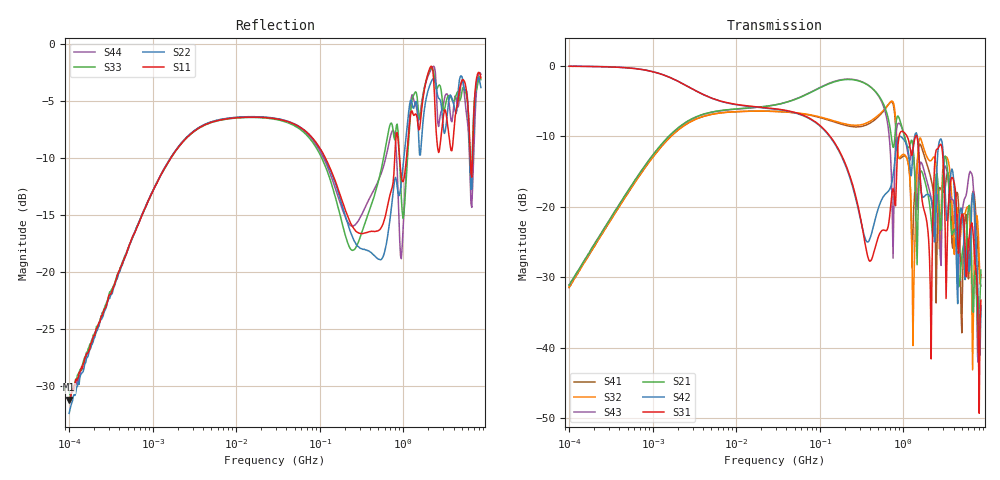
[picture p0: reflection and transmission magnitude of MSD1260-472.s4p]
# MHz S MA R 50
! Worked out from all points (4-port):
!   498 points, 100 kHz to 8.5 GHz, reference 50 ohm
!   strongest paths, dB at 100 kHz, 1.698 MHz, 29.49 MHz, 500.7 MHz, 8.5 GHz:
!     S31: -0.1, -1.8, -6.1, -24.3, -33.3
!     S42: -0.1, -1.8, -6.2, -20.3, -34.4
!     S21: -31.1, -9.6, -5.5, -4.1, -29.0
!     S43: -31.1, -9.6, -5.5, -4.2, -34.0
!     S32: -31.4, -9.9, -6.5, -7.0, -29.6
!     S41: -31.5, -9.9, -6.5, -7.3, -31.2
!   lowest |S11| = -31.2 dB at 100 kHz (marker M1), VSWR 1.06, Z = 50 + j2.77 ohm
!   |S11| at or under -10 dB: 117.4 MHz to 790.6 MHz (673.2 MHz wide, 148 % of centre); 903.2 MHz to 1.092 GHz (188.6 MHz wide, 18.9 % of centre); 6.36 GHz to 6.737 GHz (377 MHz wide, 5.76 % of centre)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
0.1  0.02766 88.8  0.02777 85.4  0.9921 -1.6  0.02665 -95.1
     0.02777 85.4  0.02411 88.8  0.02698 -95.0  0.9938 -1.6
     0.9921 -1.6  0.02698 -95.0  0.03029 90.1  0.02801 84.4
     0.02665 -95.1  0.9938 -1.6  0.02801 84.4  0.02776 92.2
3.607286  0.4304 26.0  0.4429 28.3  0.6464 -20.5  0.4275 -155.2
          0.4429 28.3  0.4324 26.1  0.4275 -155.4  0.6456 -20.8
          0.6464 -20.5  0.4275 -155.4  0.4297 26.0  0.4421 28.4
          0.4275 -155.2  0.6456 -20.8  0.4421 28.4  0.4324 26.2
241.0775  0.1616 -48.8  0.7984 -37.0  0.1513 -131.4  0.3705 49.2
          0.7984 -37.0  0.1462 -55.2  0.38 45.5  0.1463 -133.8
          0.1513 -131.4  0.38 45.5  0.1253 -31.4  0.8027 -39.9
          0.3705 49.2  0.1463 -133.8  0.8027 -39.9  0.1601 -32.6
2209.207  0.7965 168.2  0.06829 125.4  0.03688 -92.7  0.1461 101.3
          0.06829 125.4  0.6965 -170.6  0.2162 116.9  0.1051 115.3
          0.03688 -92.7  0.2162 116.9  0.7912 -179.9  0.1061 98.0
          0.1461 101.3  0.1051 115.3  0.1061 98.0  0.789 179.0
2776.003  0.3678 120.4  0.06823 74.0  0.2772 71.9  0.136 97.5
          0.06823 74.0  0.5691 112.1  0.05314 -129.4  0.3012 55.9
          0.2772 71.9  0.05314 -129.4  0.6563 103.5  0.04383 36.7
          0.136 97.5  0.3012 55.9  0.04383 36.7  0.489 111.5
6462.473  0.2719 153.6  0.0657 -22.0  0.07387 89.7  0.09171 147.0
          0.0657 -22.0  0.2302 123.3  0.04738 27.5  0.06613 134.8
          0.07387 89.7  0.04738 27.5  0.2631 127.0  0.1745 52.6
          0.09171 147.0  0.06613 134.8  0.1745 52.6  0.2009 148.9
8500  0.7136 -58.1  0.03557 -23.5  0.02171 -47.1  0.02742 -148.6
      0.03557 -23.5  0.6466 -57.9  0.0331 -127.9  0.01902 -84.2
      0.02171 -47.1  0.0331 -127.9  0.7003 -47.5  0.02001 14.1
      0.02742 -148.6  0.01902 -84.2  0.02001 14.1  0.7398 -53.5
